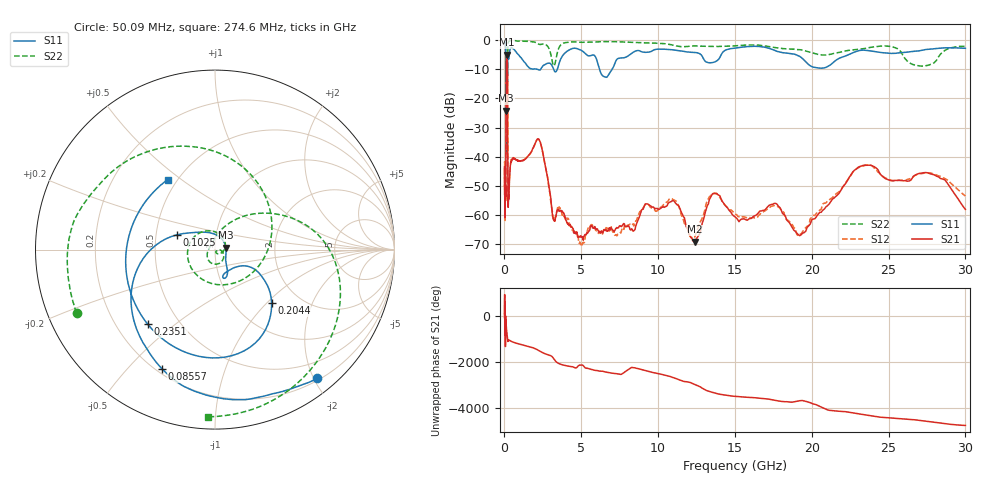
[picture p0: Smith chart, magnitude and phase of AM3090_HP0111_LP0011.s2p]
! Date/Time: Thu, Feb 28, 2019 2:00 PM
! Network Analyzer: Agilent Technologies E8364B Rev: A.07.50.67
! Sweep from 0.010 to 30.000 GHz, 1601 Points, Sweep Type: LOG
! Power Supply: 5.023 V, 0.002 A
# Hz S DB R 50
!freq MagS11 AngS11 MagS21 AngS21 MagS12 AngS12 MagS22 AngS22
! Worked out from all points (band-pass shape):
!   1601 points, 10 MHz to 30 GHz, reference 50 ohm
!   highest |S21| = -5.04 dB at 148.4 MHz (marker M1); lowest = -69.1 dB at 12.37 GHz (marker M2)
!   |S21| within 3 dB of the highest: 112.4 MHz to 189.5 MHz (77.01 MHz wide, 51 % of centre)
!   lowest |S11| = -24.2 dB at 109.9 MHz (marker M3), VSWR 1.13, Z = 56.4 + j1.31 ohm
!   |S11| at or under -10 dB: 2.138 GHz to 2.36 GHz (221.8 MHz wide, 9.86 % of centre); 3.201 GHz to 3.443 GHz (241.3 MHz wide, 7.26 % of centre); 6.184 GHz to 7.01 GHz (826.2 MHz wide, 12.5 % of centre)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
!   |S22| runs from -39.1 to -0.2 dB; largest |S21 - S12| = 0.014
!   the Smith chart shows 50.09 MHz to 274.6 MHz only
!   S11 on the Smith chart (normalised r, x): 50.09 MHz: 0.23, -2.05; 85.57 MHz: 0.22, -0.63; 102.5 MHz: 0.64, +0.11; 204.4 MHz: 1.46, -1.07; 235.1 MHz: 0.33, -0.40; 274.6 MHz: 0.44, +0.45
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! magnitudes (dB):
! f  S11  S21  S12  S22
! 10 MHz  -0.3  -44.1  -41.9  -0.5
! 38.04 MHz  -0.5  -59.1  -60.3  -1.4
! 50.09 MHz  -0.8  -51.8  -49.1  -1.4
! 85.57 MHz  -2.8  -52.2  -51.4  -5.8
! 102.5 MHz  -12.9  -16.3  -16.3  -15.1
! 109.9 MHz  -24.2  -9.1  -9.1  -17.9
! 144.7 MHz  -16.8  -5.1  -5.0  -31.0
! 148.4 MHz  -17.0  -5.0  -5.0  -26.0
! 180.3 MHz  -15.1  -6.4  -6.4  -29.7
! 204.4 MHz  -7.3  -18.1  -18.0  -9.3
! 235.1 MHz  -5.0  -56.7  -56.2  -1.4
! 274.6 MHz  -6.5  -53.8  -53.9  -0.6
! 550.5 MHz  -3.0  -40.5  -40.7  -0.3
! 2.084 GHz  -10.0  -34.5  -34.4  -1.0
! 3.22 GHz  -10.3  -61.7  -61.8  -8.9
! 7.926 GHz  -5.8  -63.9  -63.6  -0.7
! 10.92 GHz  -3.3  -55.1  -54.4  -1.7
! 12.37 GHz  -4.3  -69.1  -67.6  -2.0
! 13.74 GHz  -7.4  -52.6  -52.5  -2.2
! 19.51 GHz  -6.9  -66.0  -64.8  -3.6
! 23.48 GHz  -3.5  -42.9  -43.0  -2.9
! 30 GHz  -2.8  -58.0  -53.4  -2.2
